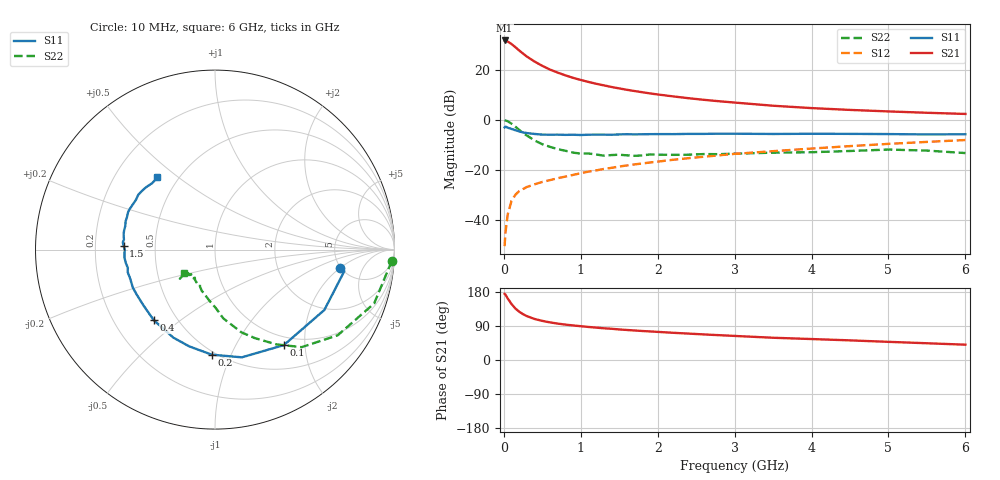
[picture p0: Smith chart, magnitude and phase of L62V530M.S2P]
!  INFINEON TECHNOLOGIES Small Signal Semiconductors
! BFR380L3 , Si-NPN RF-Transistor in TSLP-3-1
!  Vce=2.5 V,  Ic=30 mA
! Common Emitter S-Parameters:  07. March 2005
#  GHz  S  MA  R  50
! f  S11  S21  S12  S22
! GHz  Mag  Ang  Mag  Ang  Mag  Ang  Mag  Ang
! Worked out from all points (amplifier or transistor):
!   36 points, 10 MHz to 6 GHz, reference 50 ohm
!   highest |S21| = 31.7 dB at 10 MHz (marker M1)
!   |S21| within 3 dB of that: start of sweep to 161.9 MHz
!   unconditionally stable (mu >= 1): 1.695 GHz to 4.827 GHz
!   at 250 MHz: K = 0.42, MSG = 27.0 dB, |S12| = -27.6 dB
!   at 1.4 GHz: K = 0.97, MSG = 16.1 dB, |S12| = -19.2 dB
!   at 6 GHz: K = 0.98, MSG = 5.2 dB, |S12| = -8.1 dB
!   S11 on the Smith chart (normalised r, x): 10 MHz: 4.93, -1.99; 100 MHz: 0.86, -1.61; 200 MHz: 0.48, -0.85; 400 MHz: 0.37, -0.40; 1.5 GHz: 0.32, +0.02; 6 GHz: 0.39, +0.42
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0.01  0.7044 -8.3  38.27 174.5  0.003 80.0  0.9873 -3.7
0.02  0.7306 -9.4  38.1 172.9  0.0054 90.1  0.9662 -7.7
0.05  0.696 -28.9  36.5 162.5  0.0128 80.4  0.9362 -18.7
0.1  0.656 -54.2  32.47 147.7  0.0242 68.9  0.834 -34.9
0.15  0.6186 -76.0  28.1 135.9  0.0318 60.0  0.7269 -48.4
0.2  0.5856 -91.8  24.11 127.3  0.0378 57.4  0.6279 -57.2
0.25  0.5579 -104.9  20.93 120.9  0.0415 53.0  0.5403 -65.8
0.3  0.5426 -115.3  18.24 115.7  0.0455 53.3  0.4839 -72.3
0.4  0.5207 -130.9  14.49 108.2  0.0515 52.0  0.386 -83.1
0.5  0.5059 -141.4  11.92 103.2  0.0575 53.6  0.3252 -89.3
0.6  0.503 -149.3  10.04 99.2  0.0624 55.0  0.2886 -95.8
0.7  0.5046 -155.1  8.728 96.1  0.0682 56.6  0.2591 -102.2
0.9  0.5023 -165.6  6.866 91.2  0.0793 59.0  0.2212 -112.3
1.1  0.5029 -171.8  5.685 87.2  0.0922 60.9  0.2123 -118.2
1.5  0.5099 177.7  4.224 80.6  0.1165 63.2  0.2006 -128.2
1.8  0.514 171.8  3.543 76.5  0.1344 64.1  0.1937 -133.6
2.2  0.5169 165.3  2.928 71.8  0.159 64.3  0.1994 -136.5
2.8  0.5274 156.5  2.341 65.5  0.1953 64.6  0.2057 -142.7
3.5  0.5205 147.9  1.906 58.7  0.2361 62.8  0.2206 -141.5
4.5  0.5227 141.7  1.573 51.8  0.2979 61.2  0.2381 -141.0
5.5  0.5096 133.6  1.379 44.2  0.3615 57.6  0.2425 -140.7
6  0.514 128.6  1.307 40.4  0.3944 55.4  0.2165 -143.0
